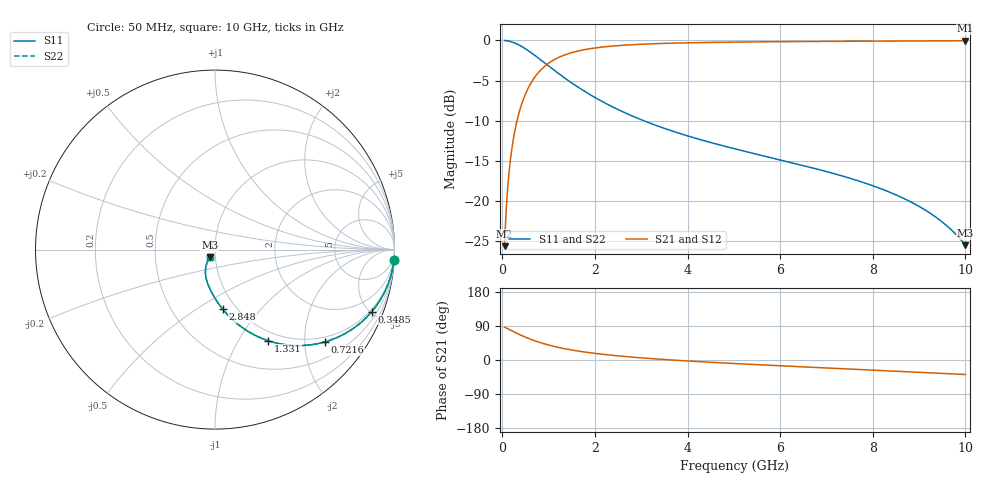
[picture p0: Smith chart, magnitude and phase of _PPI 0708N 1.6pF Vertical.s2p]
! S-Parameter data specifications (vertical orientation):
! Substrate: 40-mil Rogers 3003C, Substrate thickness, H=1.016mm, Dielectric constant, Er=3, Conductor thickness, T_mtl=0.043mm, Loss Tangent, Tand=0.003
! PCB Mounting Pad Footprint: Pad width, PadW=2.54mm , Pad length, PadL=0.51mm , Pad gap, PadG (edge-to-edge)=0.71mm , Reference planes=1.73mm apart
! Created Tue Jan 16 08:43:23 2018
# GHz S MA R 50
! 2 Port Network Data from SP1.SP block
! freq  magS11  angS11  magS21  angS21  magS12  angS12  magS22  angS22
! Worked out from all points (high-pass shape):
!   801 points, 50 MHz to 10 GHz, reference 50 ohm
!   highest |S21| = -0.05 dB at 10 GHz (marker M1); lowest = -25.6 dB at 50 MHz (marker M2)
!   |S21| within 3 dB of the highest: 953.4 MHz to end of sweep
!   lowest |S11| = -25.5 dB at 10 GHz (marker M3), VSWR 1.11, Z = 46.9 - j4.14 ohm
!   |S11| at or under -10 dB: 3.052 GHz to end of sweep
!   |S22| runs from -25.5 to 0.0 dB; largest |S21 - S12| = 0
!   S11 on the Smith chart (normalised r, x): 50 MHz: 1, -36; 348.5 MHz: 0.87, -5.11; 721.6 MHz: 0.87, -2.47; 1.331 GHz: 0.87, -1.35; 2.848 GHz: 0.87, -0.65; 10 GHz: 0.94, -0.08
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0.05  0.9986 -3.2  0.05233 86.8  0.05233 86.8  0.9986 -3.2
0.074875  0.9969 -4.8  0.07823 85.2  0.07823 85.2  0.9969 -4.8
0.124625  0.9916 -8.0  0.1295 82.0  0.1295 82.0  0.9916 -8.0
0.174375  0.9837 -11.1  0.1797 78.9  0.1797 78.9  0.9837 -11.1
0.249  0.9676 -15.7  0.2524 74.3  0.2524 74.3  0.9676 -15.7
0.3485  0.9393 -21.6  0.3427 68.4  0.3427 68.4  0.9393 -21.6
0.5101875  0.8821 -30.3  0.4707 59.7  0.4707 59.7  0.8821 -30.3
0.721625  0.7986 -40.1  0.6014 49.8  0.6014 49.8  0.7986 -40.1
1.020125  0.6859 -51.1  0.7271 38.8  0.7271 38.8  0.6859 -51.1
1.331063  0.5877 -59.7  0.8083 30.2  0.8083 30.2  0.5877 -59.7
1.716625  0.494 -67.8  0.8685 22.1  0.8685 22.1  0.494 -67.8
2.214125  0.4079 -75.4  0.9119 14.4  0.9119 14.4  0.4079 -75.4
2.848438  0.3342 -82.7  0.9412 7.1  0.9412 7.1  0.3342 -82.7
3.370812  0.2919 -87.4  0.955 2.4  0.955 2.4  0.2919 -87.4
5.025  0.2111 -99.0  0.9755 -9.4  0.9755 -9.4  0.2111 -99.0
6.691625  0.1609 -108.4  0.9845 -19.2  0.9845 -19.2  0.1609 -108.4
7.624437  0.1353 -113.4  0.988 -24.4  0.988 -24.4  0.1353 -113.4
8.345812  0.114 -117.1  0.9903 -28.5  0.9903 -28.5  0.114 -117.1
8.85575  0.09751 -119.6  0.9918 -31.4  0.9918 -31.4  0.09751 -119.6
9.291063  0.08201 -121.6  0.9929 -34.0  0.9929 -34.0  0.08201 -121.6
9.639313  0.06845 -123.0  0.9936 -36.1  0.9936 -36.1  0.06845 -123.0
10  0.05309 -124.1  0.9943 -38.3  0.9943 -38.3  0.05309 -124.1
